VAR_GLOBAL
	{attribute 'analysis' := '-33'}
	ipCreator: I_AcsiCodeCreatorClass := GVL_AcsiVars.Creator.SetCodeRev(codeRev:=8).SetGuiVer(major:=3, minor:=99, build:=5, revision:=0);
	
	(* IED data model *)
	{attribute 'analysis' := '-6'}
	fbIED: FB_IED_IED;
	{warning 'Please configure your server IP-address in the initialization code of the client function block below:'}
	(* Client connection *)
	fbIEDClient: FB_IEDClient := (fbConnection:=(ipIED:=fbIED, settings:=(sRemoteHost:='127.0.0.1', nCalled_AP_InvID:=0, nCalling_AP_InvID:=0, nCalled_AE_InvID:=0, nCalling_AE_InvID:=0)));
	
	(* Sampled values subscriber *)
	fbIED_MUnn_MSVCB01SvSubscriber: FB_IED_MUnn_MSVCB01SvSubscriber := (fbAdapter:=(ipIED:=fbIED, settings:=(eDispatchMode:=E_GseDispatchMode.NonPromiscuous)));
	fbIED_MUnn_MSVCB02SvSubscriber: FB_IED_MUnn_MSVCB02SvSubscriber := (fbAdapter:=(ipIED:=fbIED, settings:=(eDispatchMode:=E_GseDispatchMode.NonPromiscuous)));
	
	(* Critical section to secure the concurrent access to IED data from multiple tasks *)
	{attribute 'analysis' := '-6'}
	fbIEDCriticalSection: FB_IecCriticalSection;
END_VAR
VAR_GLOBAL CONSTANT
	cArrayBufferSize_IED_MUnn_LLN0_MSVCB01_Asdu1: UINT := 80; (* Max. number of buffered received samples *)
	cOversampleFactor_IED_MUnn_LLN0_MSVCB02_Asdu1: UINT := 8; (* Max. number of SV oversampling ASDUs *)
	cArrayBufferSize_IED_MUnn_LLN0_MSVCB02_Asdu1: UINT := 256; (* Max. number of buffered received samples *)
END_VAR
